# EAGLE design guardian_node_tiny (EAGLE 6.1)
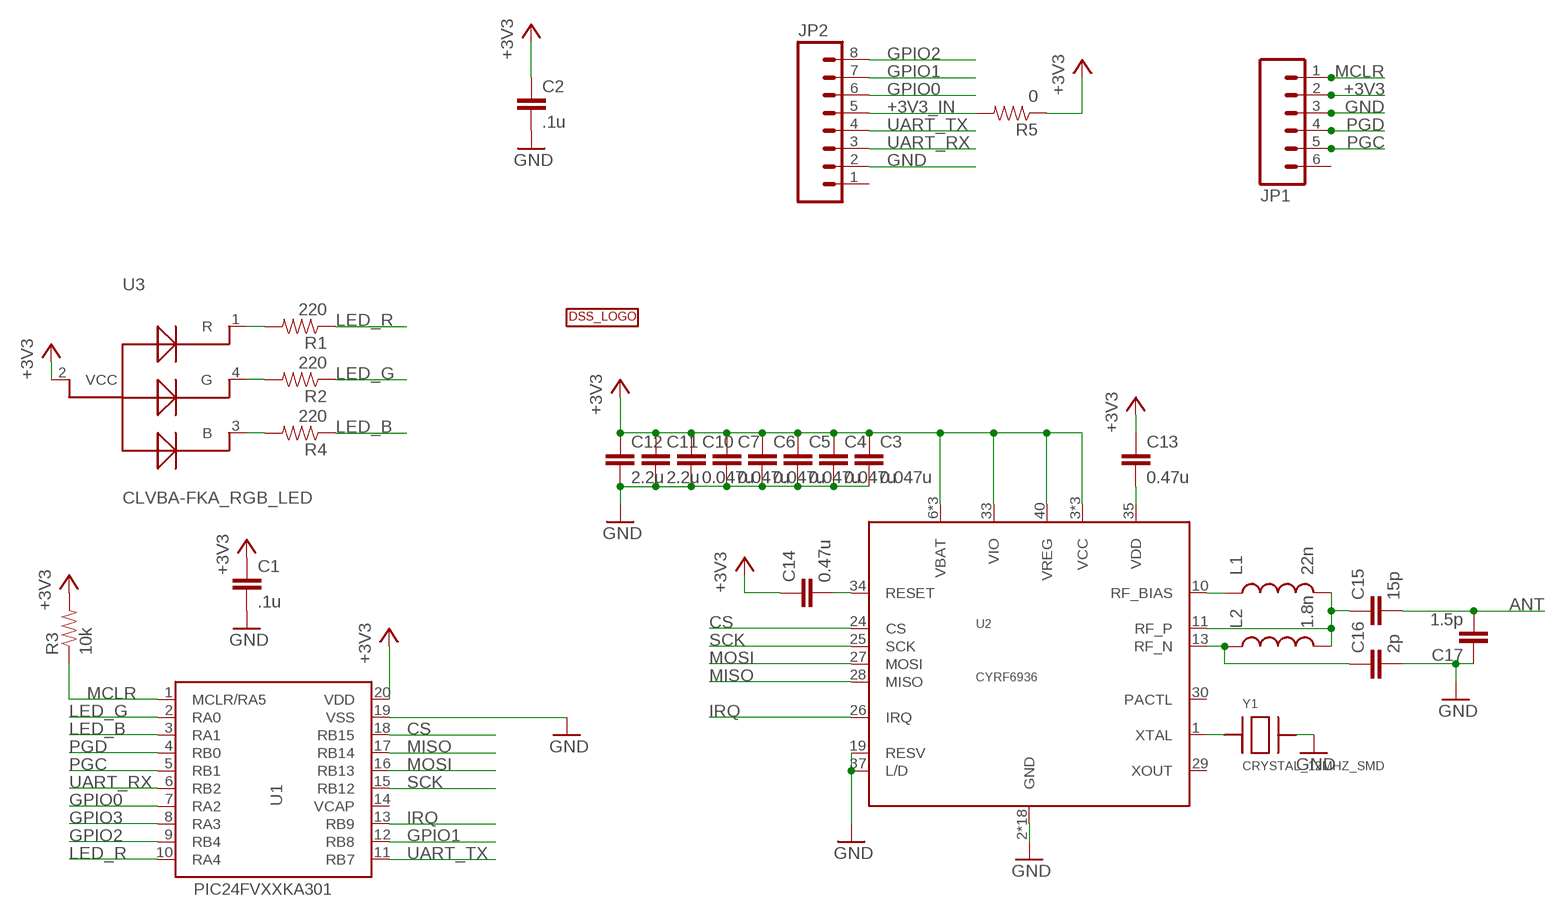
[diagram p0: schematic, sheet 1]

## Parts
C1  .1u  CAP0603-CAP  [0603-CAP]
C2  .1u  CAP0603-CAP  [0603-CAP]
C3  0.047u  CAP0402-CAP  [0402-CAP]
C4  0.047u  CAP0402-CAP  [0402-CAP]
C5  0.047u  CAP0402-CAP  [0402-CAP]
C6  0.047u  CAP0402-CAP  [0402-CAP]
C7  0.047u  CAP0402-CAP  [0402-CAP]
C10  0.047u  CAP0402-CAP  [0402-CAP]
C11  2.2u  CAP0402-CAP  [0402-CAP]
C12  2.2u  CAP0402-CAP  [0402-CAP]
C13  0.47u  CAP0402-CAP  [0402-CAP]
C14  0.47u  CAP0402-CAP  [0402-CAP]
C15  15p  CAP0402-CAP  [0402-CAP]
C16  2p  CAP0402-CAP  [0402-CAP]
C17  1.5p  CAP0402-CAP  [0402-CAP]
JP1  M06SIP  [1X06]
JP2  M081X08  [1X08]
L1  22n  INDUCTOR0603  [0603]
L2  1.8n  INDUCTOR0402  [C0402]
R1  220  RESISTOR0402-RES  [0402-RES]
R2  220  RESISTOR0402-RES  [0402-RES]
R3  10k  RESISTOR0603-RES  [0603-RES]
R4  220  RESISTOR0402-RES  [0402-RES]
R5  0  RESISTOR0603-RES  [0603-RES]
U1  PIC24FVXXKA301  [SSOP20]
U2  CYRF6936  [QFN40-6X6]
U3  CLVBA-FKA_RGB_LED  [PLCC-4]
U$1  DSSBOTTOM  [DSS_BOT]
Y1  CRYSTAL_12MHZ_SMD  [SMD-4_5X3.2MM]

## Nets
+3V3: C1.1 C2.1 C3.1 C4.1 C5.1 C6.1 C7.1 C10.1 C11.1 C12.1 C13.1 C14.1 JP1.2 R3.2 R5.1 U1.20(VDD) U2.3(VCC) U2.6(VBAT) U2.7(VCC) U2.8(VBAT) U2.16(VCC) U2.33(VIO) U2.38(VBAT) U2.40(VREG) U3.2(VCC)
+3V3_IN: JP2.5 R5.2
ANT: C15.2 C17.2
CS: U1.18(RB15) U2.24(CS)
GND: C1.2 C2.2 C3.2 C4.2 C5.2 C6.2 C7.2 C10.2 C11.2 C12.2 C16.2 C17.1 JP1.3 JP2.2 U1.19(VSS) U2.2(GND) U2.4(GND) U2.5(GND) U2.9(GND) U2.12(GND) U2.14(GND) U2.15(GND) U2.17(GND) U2.18(GND) U2.19(RESV) U2.20(GND) U2.21(GND) U2.22(GND) U2.23(GND) U2.31(GND) U2.32(GND) U2.36(GND) U2.37(L/D) U2.39(GND) U2.EXP(GND) Y1.P$3
GPIO0: JP2.6 U1.7(RA2)
GPIO1: JP2.7 U1.12(RB8)
GPIO2: JP2.8 U1.9(RB4)
GPIO3: U1.8(RA3)
IRQ: U1.13(RB9) U2.26(IRQ)
LED_B: R4.1 U1.3(RA1)
LED_G: R2.1 U1.2(RA0)
LED_R: R1.1 U1.10(RA4)
MCLR: JP1.1 R3.1 U1.1(MCLR/RA5)
MISO: U1.17(RB14) U2.28(MISO)
MOSI: U1.16(RB13) U2.27(MOSI)
N$1: R1.2 U3.1(R)
N$2: R2.2 U3.4(G)
N$3: R4.2 U3.3(B)
N$5: L1.1 U2.10(RF_BIAS)
N$6: C15.1 L1.2 L2.2 U2.11(RF_P)
N$7: C13.2 U2.35(VDD)
N$8: C14.2 U2.34(RESET)
N$9: C16.1 L2.1 U2.13(RF_N)
N$10: U2.1(XTAL) Y1.P$1
PGC: JP1.5 U1.5(RB1)
PGD: JP1.4 U1.4(RB0)
SCK: U1.15(RB12) U2.25(SCK)
UART_RX: JP2.3 U1.6(RB2)
UART_TX: JP2.4 U1.11(RB7)
Unconnected: JP1.6 JP2.1 U1.14(VCAP) U2.29(XOUT) U2.30(PACTL)

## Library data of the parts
C1-C7 C10-C17 = SparkFun-Passives:CAP: Capacitor
JP1 = SparkFun-Connectors:M06: Header 6 Standard 6-pin 0.1" header. Use with straight break away headers (SKU : PRT-00116), right angle break away headers (PRT-00553), swiss pins (PRT-00743), machine pins (PRT-00117), and female headers (PRT-00115). Molex polarized connector foot print use with SKU : PRT-08094 with associated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
JP2 = SparkFun-Connectors:M08: Header 8 Standard 8-pin 0.1" header. Use with straight break away headers (SKU : PRT-00116), right angle break away headers (PRT-00553), swiss pins (PRT-00743), machine pins (PRT-00117), and female headers (PRT-00115).
L1 L2 = SparkFun-Passives:INDUCTOR: Inductors
R1-R5 = SparkFun-Passives:RESISTOR: Resistor
U1 = DSS:PIC24FVXXKA301: PIC24FVXXKA301
U2 = DSS:CYRF6936: Cypress CYRF6936 2.4GHz DSSS radio. All N/C pins and the exposed pad are tied to ground.
U3 = DSS:CLVBA-FKA_RGB_LED
U$1 = DSS:DSS: DSS LOGO
Y1 = DSS:CRYSTAL_12MHZ_SMD: 12MHz crystal, SMD

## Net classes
2 VCC: width 0.406 mm, clearance 0.381 mm

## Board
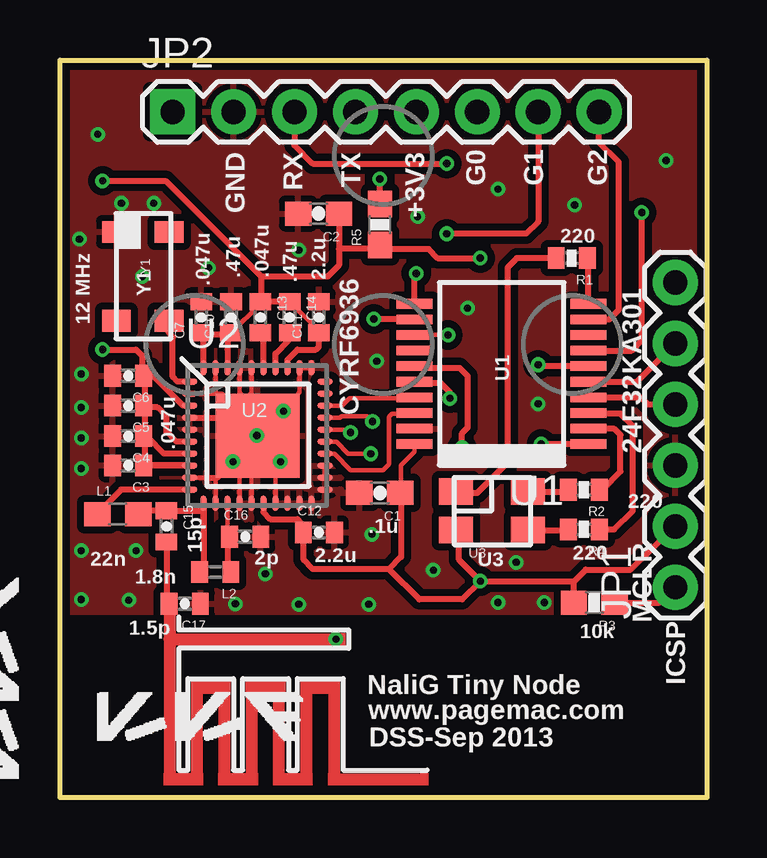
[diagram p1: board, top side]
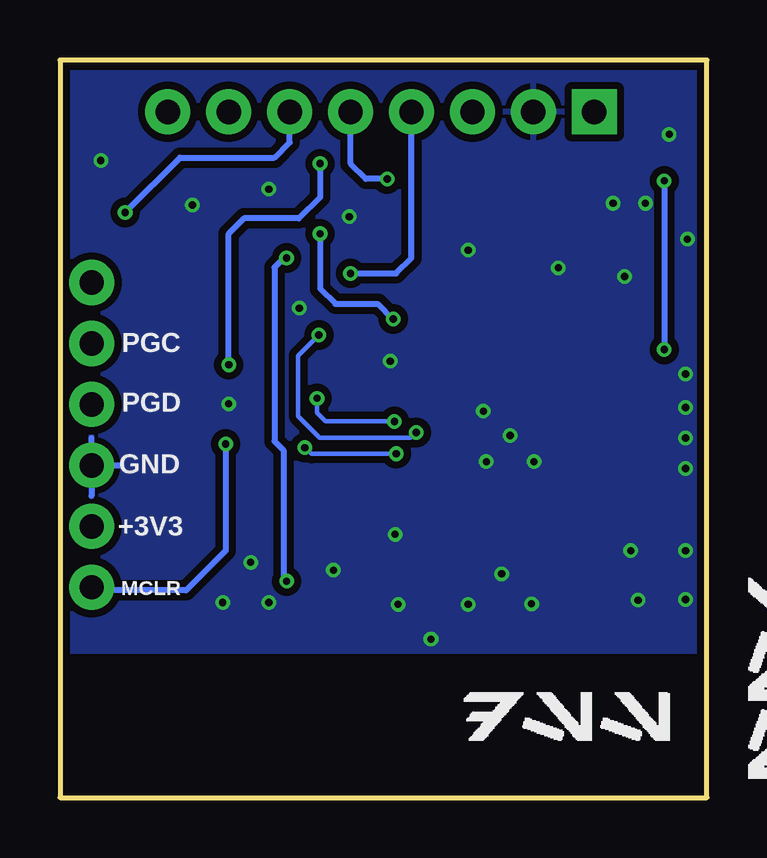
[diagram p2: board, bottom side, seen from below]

Size 26.97 x 30.73 mm. Coordinates in mm from the lower left corner, seen from the top.
Outline: 0,30.73 26.98,30.73 26.98,0 0,0 0,30.73
Copper layers (1*16): Top 0.035mm / dielectric 1.5mm / Bottom 0.035mm
Design rules: minimum track width 6mil, minimum drill 12mil, track to track 6mil, track to pad 6mil, pad to pad 6mil, via to via 6mil, smd to smd 0mil, copper to edge 10mil, drill to drill 10mil, minimum pad ring 10mil, minimum via ring 6mil, stop-mask expansion 2mil, vias tented up to drill 100mil, thermal gap 10mil

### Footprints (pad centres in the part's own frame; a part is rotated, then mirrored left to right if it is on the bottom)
0603-CAP = smd 1.1 x 1: 1 -0.85,0; 2 0.85,0
0402-CAP = smd 0.7 x 0.9: 1 -0.65,0; 2 0.65,0
1X06 = drill 1.016 pad 1.88: 1 0,0; 2 2.54,0; 3 5.08,0; 4 7.62,0; 5 10.16,0; 6 12.7,0
1X08 = drill 1.016 pad 1.88 square: 1 0,0 | drill 1.016 pad 1.88: 2 2.54,0; 3 5.08,0; 4 7.62,0; 5 10.16,0; 6 12.7,0; 7 15.24,0; 8 17.78,0
0603 = smd 1.1 x 1: 1 -0.85,0; 2 0.85,0
C0402 = smd 0.7 x 0.9: 1 -0.65,0; 2 0.65,0
0402-RES = smd 0.7 x 0.9: 1 -0.65,0; 2 0.65,0
0603-RES = smd 1.1 x 1: 1 -0.85,0; 2 0.85,0
SSOP20 = smd 0.4 x 1.5: 1 -2.925,-3.625; 2 -2.275,-3.625; 3 -1.625,-3.625; 4 -0.975,-3.625; 5 -0.325,-3.625; 6 0.325,-3.625; 7 0.975,-3.625; 8 1.625,-3.625; 9 2.275,-3.625; 10 2.925,-3.625; 11 2.925,3.625; 12 2.275,3.625; 13 1.625,3.625; 14 0.975,3.625; 15 0.325,3.625; 16 -0.325,3.625; 17 -0.975,3.625; 18 -1.625,3.625; 19 -2.275,3.625; 20 -2.925,3.625
QFN40-6X6 = smd 0.65 x 0.25: 1 -2.825,2.25; 2 -2.825,1.75; 3 -2.825,1.25; 4 -2.825,0.75; 5 -2.825,0.25; 6 -2.825,-0.25; 7 -2.825,-0.75; 8 -2.825,-1.25; 9 -2.825,-1.75; 10 -2.825,-2.25; 21 2.825,-2.25; 22 2.825,-1.75; 23 2.825,-1.25; 24 2.825,-0.75; 25 2.825,-0.25; 26 2.825,0.25; 27 2.825,0.75; 28 2.825,1.25; 29 2.825,1.75; 30 2.825,2.25 | smd 0.25 x 0.65: 11 -2.25,-2.825; 12 -1.75,-2.825; 13 -1.25,-2.825; 14 -0.75,-2.825; 15 -0.25,-2.825; 16 0.25,-2.825; 17 0.75,-2.825; 18 1.25,-2.825; 19 1.75,-2.825; 20 2.25,-2.825; 31 2.25,2.825; 32 1.75,2.825; 33 1.25,2.825; 34 0.75,2.825; 35 0.25,2.825; 36 -0.25,2.825; 37 -0.75,2.825; 38 -1.25,2.825; 39 -1.75,2.825; 40 -2.25,2.825 | smd 3.5 x 3.5: EXP 0,0
PLCC-4 = smd 1.4 x 1.1: 1 -1.524,0.812; 2 -1.524,-0.788; 3 1.476,-0.788; 4 1.476,0.812
SMD-4_5X3.2MM = smd 0.9 x 1.2: P$1 1.9,1.1; P$2 1.9,-1.1; P$3 -1.8,-1.1; P$4 -1.8,1.1

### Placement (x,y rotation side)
C1  13.34,12.7 180 top
C2  10.78,24.34 180 top
C3  2.84,13.84 180 top
C4  2.84,15.06 180 top
C5  2.84,16.33 180 top
C6  2.84,17.58 180 top
C7  5.89,20.02 90 top
C10  7.14,20.02 90 top
C11  10.79,20.02 90 top
C12  10.79,11.05 0 top
C13  8.36,20.02 270 top
C14  9.58,20.02 270 top
C15  4.45,11.3 270 top
C16  7.72,10.87 0 top
C17  5.21,8.08 180 top
JP1  25.65,8.76 90 top
JP2  4.7,28.57 0 top
L1  2.41,11.81 0 top
L2  6.48,9.4 180 top
R1  21.34,22.48 180 top
R2  21.84,12.83 180 top
R3  22.28,8.13 180 top
R4  21.84,11.18 180 top
R5  13.34,23.88 90 top
U1  18.41,17.65 90 top
U2  8.23,15.09 0 top
U3  18.03,11.94 0 top
U$1  -1.52,0.64 90 top
Y1  3.45,21.77 270 top

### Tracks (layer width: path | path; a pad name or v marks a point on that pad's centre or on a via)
+3V3  (via drill 0.3)
  Top 0.178: U2.33 9.49,17.91 9.53,17.88 | 10.79,19.45 C14.1 | 8.36,20.58 C10.1 | U1.20 14.79,14.41 14.22,13.84 14.22,12.74 C1.1 | 10.16,11.3 C12.1
  Top 0.254: 3.56,13.84 U2.8 3.56,13.84 | U2.7 4.33,14.34 3.68,14.99 3.57,14.99 C4.1 3.55,15.11 3.56,15.11 | 3.43,16.39 C5.1 | U2.38 6.99,18.67 7.01,19.46 C10.1 7.08,19.3 5.97,19.3 5.98,19.29 U2.40 5.98,19.17 5.84,19.3 5.89,19.36 C7.1 | U2.16 8.48,11.89 8.76,11.61 9.91,11.61 10.16,11.3 | 10.79,19.45 C11.1 10.79,18.8 10.67,18.67 9.91,18.67 9.48,18.24 U2.33 | C14.1 C13.1 | C13.1 8.36,20.58 | 8.38,20.64 8.38,21.72 8.4,21.7 | v1.78,18.67 3.17,18.67 3.43,18.41 3.43,17.64 C6.1 3.55,17.53 3.56,17.53 | U2.6 4.85,14.84 4.45,15.24 4.45,15.88 4.06,16.26 3.43,16.26 3.43,16.27 C5.1 | U2.3 5.12,16.34 3.94,17.53 3.56,17.53 | 3.43,13.72 3.56,13.84 | C3.1 3.56,13.84 | 3.56,13.84 3.56,15.11 | 3.56,15.11 3.56,16.38 | 3.56,16.38 3.56,17.53 | C5.1 3.5,16.33 3.56,16.38 | 8.38,20.57 8.38,20.64 | 8.38,20.64 C13.1 | 16.41,11.05 U3.2 | R3.2 21.42,9 | 21.42,9 21.92,9.5 23.8,9.5 JP1.2 | 21.42,9 17.54,9 v17.53,9.02 | v17.53,9.02 16.64,9.91 16.64,11.02 U3.2 | 16.48,11.18 U3.2 | 14.22,12.74 14.22,10.03 13.72,9.53 | v17.53,9.02 16.76,8.26 14.99,8.26 13.72,9.53 | v1.78,25.7 4.4,25.7 8.4,21.7 | 8.4,21.7 8.42,21.72 11.18,21.72 11.63,22.18 11.63,22.86 | C2.1 11.63,22.86 | 11.63,22.86 13.17,22.86 R5.1 13.34,22.86 15.37,22.86 15.75,22.48 v17.53,22.48 | 13.72,9.53 10.54,9.53 10.16,9.91 10.16,11.05 C12.1
  Bottom 0.254: v1.78,25.7 v1.78,18.67 | v17.53,9.02 17.65,9.14 17.65,14.48 18.03,14.86 18.03,22.1 17.65,22.48 v17.53,22.48
+3V3_IN  (via drill 0.3)
  Top 0.254: R5.2 v13.34,25.78
  Bottom 0.254: v13.34,25.78 14.22,25.78 14.86,26.42 JP2.5
ANT
  Top 0.254: C15.2 4.45,8.29 C17.2
CS
  Top 0.178: U2.24 11.44,14.34 12.12,13.64 13.46,13.64 13.72,13.89 13.72,15.88 13.84,16 14.76,16
  Top 0.254: 14.76,16 U1.18
GND  (via drill 0.3)
  Top 0.178: U2.9 6.1,13.34 | U2.12 6.48,13.26 6.83,13.61 v7.21,13.99 | U2.17 8.98,13.51 | 8.98,13.51 8.98,13.91 v9.2,13.99 | U2.15 7.98,13.41 8.05,13.49 8.05,13.41 8.88,13.41 8.98,13.51 | U2.14 7.48,13.73 | 6.95,15.84 7.44,15.82 | U2.2 6.53,16.84 | 6.53,16.84 6.76,16.84 7.01,16.59 7.01,16.26 7.44,15.82 | U2.39 6.48,16.89 6.53,16.84 | U2.37 7.48,16.88 7.62,16.74 7.62,16.48 7.24,16.1 | U2.36 7.98,16.87 7.24,16.13 7.44,15.82 | U2.32 9.98,16.89 v9.32,16.1 | 10.01,17.91 U2.31 | U2.31 | U2.31 | U2.23 U2.22
  Top 0.254: U2.4 6.95,15.84 7.24,16.13 | 6.1,13.34 6.56,13.34 6.83,13.61 | 7.44,15.82 7.47,15.82 v8.2,15.09
  Top 0.508: 4.57,8.26 4.57,6.6 | 4.57,6.6 4.57,0.76 5.71,0.76 5.71,4.57 6.86,4.57 6.86,0.76 | 4.57,6.6 v11.51,6.6 11.66,6.6
  Bottom 0.254: JP1.3 24.43,13.84 | JP1.3 25.65,14.99 | JP1.3 25.65,12.57
  other vias: 3.91,24.77 9.96,8.05 6.2,22.07 15.57,9.47 0.89,17.65 7.32,8.08 0.89,8.26 0.89,10.29 2.87,8.23 13.21,18.19 0.89,16.26 0.89,14.99 0.89,13.72 3.17,10.29 18.26,8.13 20.19,8.13 0.81,23.27 3.43,21.72 2.57,24.77 19.02,9.8 18.26,25.35 21.45,24.69 25.27,26.54 14.91,24.21 1.57,27.64 19.94,16.41 12.88,8.05 9.96,22.81 16.99,20.4 8.56,9.32 13,10.97
  pour Bottom (isolate 0.305): 0,6.07 26.92,6.07 26.92,30.35 0.03,30.3
  pour Top (isolate 0.305): 0,7.72 27.05,7.72 27.05,30.35 0.15,30.3
GPIO0  (via drill 0.3)
  Top 0.254: U1.7 23.84,18.63 24.26,19.05 v24.26,24.38
  Bottom 0.254: v24.26,24.38 21.97,26.67 18.03,26.67 17.4,27.3 JP2.6
GPIO1  (via drill 0.3)
  Top 0.254: U1.12 13.09,19.93 v13.08,19.94 | JP2.7 19.94,24 19.43,23.5 v16.13,23.5
  Bottom 0.254: v16.13,23.5 16.13,21.21 15.49,20.57 13.72,20.57 v13.08,19.94
GPIO2
  Top 0.254: U1.9 22.9,19.93 23.29,20.32 23.29,26.49 22.48,27.3 JP2.8
IRQ  (via drill 0.3)
  Top 0.178: U2.26 11.99,15.34 v12.12,15.21 | U1.13 v16.18,19.28
  Bottom 0.178: v12.12,15.21 12.37,14.99 16.15,14.99 17.04,15.9 17.04,18.41 v16.18,19.28
LED_B
  Top 0.254: R4.1 23.11,11.18 23.88,11.94 23.88,15.49 23.37,16 22.07,16 U1.3
LED_G
  Top 0.254: R2.1 22.61,12.83 23.37,13.59 23.37,15.11 23.11,15.37 22.05,15.37 U1.2
LED_R
  Top 0.254: U1.10 22.04,22.43 R1.1
MCLR  (via drill 0.3)
  Top 0.254: U1.1 v20.07,14.73 | R3.1 24.99,8.13 JP1.1
  Bottom 0.254: v20.07,14.73 20.07,10.29 21.72,8.64 25.53,8.64 JP1.1
MISO
  Top 0.178: U2.28 11.77,16.34 12.06,16.64 14.75,16.64
  Top 0.254: 14.75,16.64 U1.17
MOSI  (via drill 0.3)
  Top 0.178: U2.27 11.67,15.84 11.73,15.9 12.8,15.9 v13.03,15.67
  Top 0.254: U1.16 14.85,17.27 14.86,17.27 15.88,17.27 16.26,16.89 v16.26,16.64
  Bottom 0.178: v13.03,15.67 15.9,15.67 16.26,16.03 v16.26,16.64
N$1
  Top 0.178: 16.56,12.7 U3.1
  Top 0.254: R1.2 19.05,22.48 18.67,22.1 18.67,13.97 17.4,12.7 16.56,12.7
N$2
  Top 0.254: U3.4 21.37,12.75 R2.2
N$3
  Top 0.254: U3.3 21.42,11.15 R4.2
N$5
  Top 0.254: U2.10 2.55,12.84 1.4,11.68 1.4,11.72 L1.1
N$6
  Top 0.254: U2.11 5.98,11.05 | 5.98,11.05 5.98,9.54 5.84,9.4 L2.2 | 5.98,11.05 5.96,11.95 C15.1 3.15,11.95 L1.2
N$7
  Top 0.254: U2.35 8.48,19.24 C13.2
N$8
  Top 0.254: U2.34 8.98,18.5 9.53,19.05 9.53,19.31 C14.2
N$9
  Top 0.178: U2.13 6.97,10.48
  Top 0.254: 6.97,10.48 C16.1 7.01,10.49 | L2.1 7.01,9.53 7.01,10.49 | 7.01,10.49 7.01,10.54 | 7.01,10.54 7.01,10.49 | 7.01,10.49 7.01,10.54
N$10
  Top 0.254: U2.1 4.89,17.34 4.7,17.53 4.7,19.18 4.32,19.68 4.57,19.81 4.55,19.92 Y1.P$1
N$11
  Top 0.508: 6.86,0.76 8,0.76 8,4.57 9.14,4.57 9.14,0.76
N$12
  Top 0.508: 9.14,0.76 10.29,0.76 10.29,4.57 11.43,4.57 11.43,0.76 15.11,0.76
PGC
  Top 0.254: U1.5 24.06,17.33 JP1.5
PGD
  Top 0.254: U1.4 24.22,16.68 24.51,16.38 JP1.4
SCK  (via drill 0.3)
  Top 0.178: U2.25 11.53,14.84 12.01,14.33 v12.95,14.33
  Top 0.254: U1.15 14.86,17.91 16.66,17.91 16.99,17.58 16.99,15.42 16.76,15.19 v16.76,14.58
  Bottom 0.178: v12.95,14.33 16.48,14.33 16.64,14.48 v16.76,14.58
UART_RX  (via drill 0.3)
  Top 0.254: U1.6 19.94,17.98 v19.94,18.03 | JP2.3 9.78,27.18 10.54,26.42 v16.13,26.42
  Bottom 0.254: v19.94,18.03 19.94,23.5 19.3,24.13 17.02,24.13 16.13,25.02 v16.13,26.42
UART_TX  (via drill 0.3)
  Top 0.254: U1.11 14.79,21.65 v14.86,21.84
  Bottom 0.254: v14.86,21.84 12.95,21.84 12.32,22.48 JP2.4
(copper drawn outside any net)
  shapes: Top area x9

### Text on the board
tDocu: B0 | B3 | B4 | B2 | B1
_tsilk: GND | RX | TX | +3V3 | G0 | G1 | G2 | .047u | 220 | 12 MHz | .47u | Y1 | 2.2u | .047u | .47u | 24F32KA301 | U1 | .047u | U2 | CYRF6936 | 220 | 15p | .1u | 220 | 22n | 1.8n | 2p | 2.2u | U3 | 1.5p | 10k | MCLR | ICSP | NaliG Tiny Node | www.pagemac.com | DSS-Sep 2013
_bsilk: PGC | PGD | GND | +3V3 | MCLR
